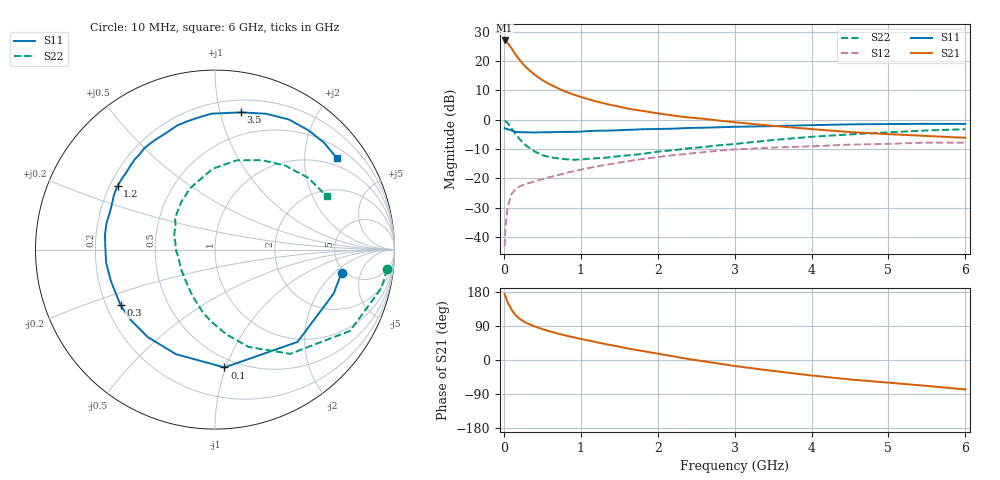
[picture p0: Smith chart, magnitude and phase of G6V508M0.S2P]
! SIEMENS Small Signal Semiconductors
! BFG193
! Si NPN RF Bipolar Junction Transistor in SOT223
! VCE = 0.5 V  IC = 8 mA
! Common Emitter S-Parameters:  August  1996
# GHz  S  MA  R  50
!  f  S11  S21  S12  S22
! GHz  MAG  ANG  MAG  ANG  MAG  ANG  MAG  ANG
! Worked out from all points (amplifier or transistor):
!   36 points, 10 MHz to 6 GHz, reference 50 ohm
!   highest |S21| = 27.0 dB at 10 MHz (marker M1)
!   |S21| within 3 dB of that: start of sweep to 108 MHz
!   unconditionally stable (mu >= 1): 840.1 MHz to 4.444 GHz; 5.758 GHz to end of sweep
!   at 250 MHz: K = 0.49, MSG = 20.6 dB, |S12| = -22.3 dB
!   at 1.4 GHz: K = 1.11, MAG = 8.0 dB, |S12| = -15.1 dB
!   at 6 GHz: K = 1.01, MAG = 0.3 dB, |S12| = -7.8 dB
!   S11 on the Smith chart (normalised r, x): 10 MHz: 4.69, -2.50; 100 MHz: 0.43, -0.99; 300 MHz: 0.26, -0.26; 1.2 GHz: 0.23, +0.28; 3.5 GHz: 0.30, +1.16; 6 GHz: 0.77, +2.82
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0.01  0.7172 -10.4  22.44 174.0  0.007 86.7  0.9656 -6.5
0.02  0.7047 -20.4  22.17 169.0  0.0141 79.3  0.9517 -13.0
0.05  0.6899 -48.2  20.4 152.0  0.0329 67.3  0.8786 -31.0
0.1  0.6586 -85.4  16.5 132.9  0.0542 53.5  0.7162 -54.2
0.15  0.622 -110.5  13.01 118.6  0.0652 44.7  0.5734 -71.0
0.2  0.6147 -127.5  10.67 109.7  0.0722 40.7  0.4759 -82.4
0.25  0.6119 -140.2  8.871 102.4  0.0771 38.0  0.401 -93.2
0.3  0.6108 -149.5  7.583 97.0  0.0814 37.5  0.3539 -101.3
0.4  0.6061 -163.3  5.852 88.8  0.0892 36.9  0.2878 -115.7
0.5  0.611 -173.3  4.732 81.5  0.0967 36.8  0.2494 -127.9
0.6  0.6112 178.8  3.99 75.5  0.1057 37.4  0.2301 -138.3
0.7  0.6189 172.1  3.448 69.8  0.1136 37.6  0.2198 -147.8
0.8  0.622 166.2  3.02 64.8  0.1226 37.3  0.2127 -156.9
1.1  0.6405 151.5  2.23 51.3  0.1496 36.1  0.2161 -177.7
1.2  0.6487 146.8  2.058 47.2  0.159 35.5  0.2203 175.9
1.6  0.6727 131.8  1.559 30.9  0.1955 29.8  0.2463 156.2
2.2  0.7042 112.8  1.18 9.8  0.2482 18.8  0.3015 133.0
2.8  0.7441 96.1  0.965 -9.6  0.2977 6.3  0.367 112.8
3.5  0.778 79.3  0.786 -28.8  0.3354 -10.1  0.4512 91.5
4.5  0.8335 60.5  0.616 -51.3  0.3766 -28.6  0.5625 62.4
5.5  0.8509 44.5  0.529 -68.4  0.408 -50.2  0.6561 37.4
6  0.8489 36.8  0.492 -77.7  0.4069 -62.7  0.6895 25.5
